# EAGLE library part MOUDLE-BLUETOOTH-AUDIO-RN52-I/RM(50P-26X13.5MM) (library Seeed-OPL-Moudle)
317030023
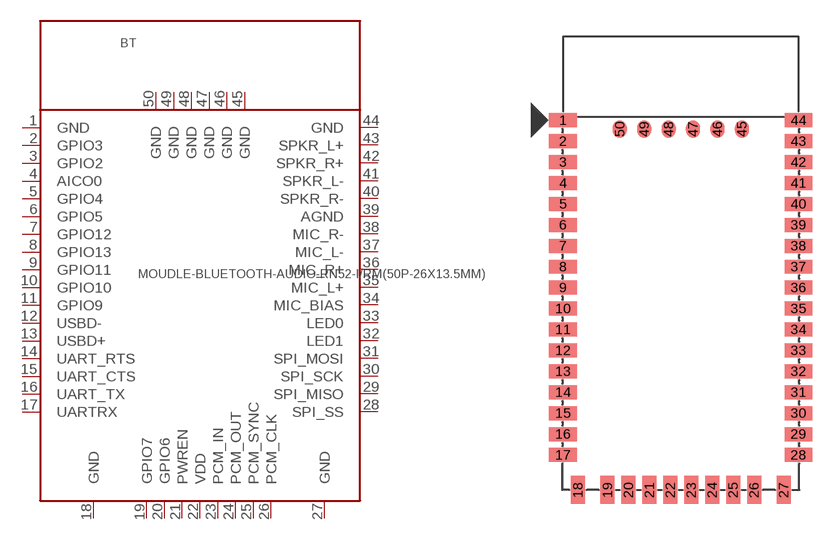
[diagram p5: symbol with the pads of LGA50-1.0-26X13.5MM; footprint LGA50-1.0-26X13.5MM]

Designator prefix BT

## MOUDLE-BLUETOOTH-AUDIO-RN52-I/RM(50P-26X13.5MM) (MPN: RN52-I/RM; VALUE: RN52-I/RM)  [LGA50-1.0-26X13.5MM]
1  GND
2  GPIO3
3  GPIO2
4  AICO0
5  GPIO4
6  GPIO5
7  GPIO12
8  GPIO13
9  GPIO11
10  GPIO10
11  GPIO9
12  USBD-
13  USBD+
14  UART_RTS
15  UART_CTS
16  UART_TX
17  UARTRX
18  GND
19  GPIO7
20  GPIO6
21  PWREN
22  VDD
23  PCM_IN
24  PCM_OUT
25  PCM_SYNC
26  PCM_CLK
27  GND
28  SPI_SS
29  SPI_MISO
30  SPI_SCK
31  SPI_MOSI
32  LED1
33  LED0
34  MIC_BIAS
35  MIC_L+
36  MIC_R+
37  MIC_L-
38  MIC_R-
39  AGND
40  SPKR_R-
41  SPKR_L-
42  SPKR_R+
43  SPKR_L+
44  GND
45  GND
46  GND
47  GND
48  GND
49  GND
50  GND

## Footprint LGA50-1.0-26X13.5MM (pad centres in mm)
smd 1.6 x 0.8: 1 -6.75,8.2; 2 -6.75,7; 3 -6.75,5.8; 4 -6.75,4.6; 5 -6.75,3.4; 6 -6.75,2.2; 7 -6.75,1; 8 -6.75,-0.2; 9 -6.75,-1.4; 10 -6.75,-2.6; 11 -6.75,-3.8; 12 -6.75,-5; 13 -6.75,-6.2; 14 -6.75,-7.4; 15 -6.75,-8.6; 16 -6.75,-9.8; 17 -6.75,-11; 28 6.75,-11; 29 6.75,-9.8; 30 6.75,-8.6; 31 6.75,-7.4; 32 6.75,-6.2; 33 6.75,-5; 34 6.75,-3.8; 35 6.75,-2.6; 36 6.75,-1.4; 37 6.75,-0.2; 38 6.75,1; 39 6.75,2.2; 40 6.75,3.4; 41 6.75,4.6; 42 6.75,5.8; 43 6.75,7; 44 6.75,8.2
smd 0.8 x 1.6: 18 -5.9,-13; 19 -4.2,-13; 20 -3,-13; 21 -1.8,-13; 22 -0.6,-13; 23 0.6,-13; 24 1.8,-13; 25 3,-13; 26 4.2,-13; 27 5.9,-13
smd 0.8 x 1: 45 3.5,7.7; 46 2.1,7.7; 47 0.7,7.7; 48 -0.7,7.7; 49 -2.1,7.7; 50 -3.5,7.7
